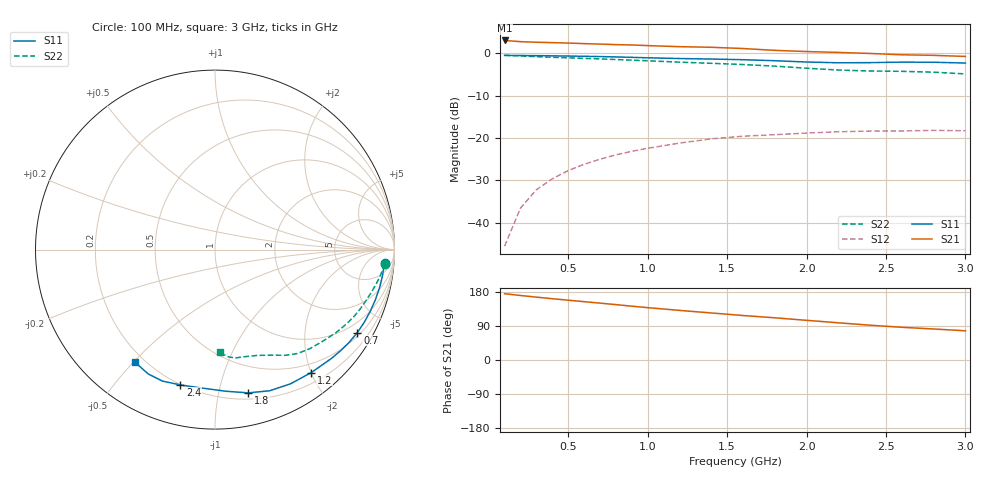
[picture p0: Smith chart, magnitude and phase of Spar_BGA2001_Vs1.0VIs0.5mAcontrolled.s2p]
! Filename: 1_5G1.001
! Title: BGA2001 X0297-20 HFE=80
! Bias: Vce=1V; Ic=.5mA controlled
! Company: NXP Semiconductors NL
! User: Quality&Reliability T&D
! Measure time: 23 Oct 1998 / 08:33:08
#  MHz  S  MA  R 50
! Freq  S11  S21  S12  S22  :
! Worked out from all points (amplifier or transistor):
!   20 points, 100 MHz to 3 GHz, reference 50 ohm
!   highest |S21| = 3.1 dB at 100 MHz (marker M1)
!   |S21| within 3 dB of that: start of sweep to 2.337 GHz
!   unconditionally stable (mu >= 1): start of sweep to 109.8 MHz
!   at 400 MHz: K = 0.26, MSG = 16.1 dB, |S12| = -29.6 dB
!   at 1.2 GHz: K = 0.40, MSG = 11.4 dB, |S12| = -21.2 dB
!   at 3 GHz: K = 0.99, MSG = 8.8 dB, |S12| = -18.3 dB
!   lowest NFmin = 1.33 dB at 1.8 GHz
!   S11 on the Smith chart (normalised r, x): 100 MHz: 12, -17; 700 MHz: 0.61, -3.61; 1.2 GHz: 0.35, -2.00; 1.8 GHz: 0.25, -1.23; 2.4 GHz: 0.20, -0.76; 3 GHz: 0.16, -0.51
100  0.9471 -4.4  1.423 174.9  0.00526 52.8  0.9494 -4.8
200  0.9448 -8.7  1.377 170.3  0.01484 84.0  0.933 -8.9
300  0.9412 -13.1  1.356 165.9  0.02445 80.6  0.9161 -12.5
400  0.9362 -17.4  1.341 161.7  0.03295 77.1  0.9 -15.9
500  0.9309 -21.7  1.326 157.8  0.04113 74.1  0.8861 -19.1
600  0.925 -26.0  1.306 153.9  0.04888 71.1  0.8739 -22.3
700  0.918 -30.2  1.289 150.1  0.05613 68.2  0.8614 -25.3
800  0.9091 -34.5  1.27 146.2  0.06314 65.3  0.8469 -28.3
900  0.8985 -38.8  1.259 142.0  0.06951 62.4  0.8324 -31.3
1000  0.888 -43.1  1.237 138.2  0.07555 59.7  0.8183 -34.3
1200  0.8702 -51.9  1.202 130.9  0.08697 54.3  0.7882 -40.3
1400  0.8579 -60.7  1.182 124.2  0.09768 49.3  0.7641 -46.2
1600  0.8431 -68.9  1.142 117.4  0.105 44.9  0.7394 -51.5
1800  0.8197 -76.9  1.087 111.4  0.1094 41.4  0.7075 -56.4
2000  0.7917 -85.5  1.052 104.7  0.1144 36.7  0.6686 -61.6
2200  0.7749 -95.2  1.027 98.2  0.1185 31.8  0.6362 -67.9
2400  0.7782 -104.3  0.9987 91.8  0.1208 28.0  0.6195 -74.4
2600  0.7889 -111.8  0.9638 86.3  0.1211 26.0  0.614 -79.6
2800  0.7862 -118.3  0.9488 81.8  0.123 23.1  0.6002 -83.4
3000  0.7698 -125.2  0.9212 77.1  0.1217 20.8  0.5725 -87.4
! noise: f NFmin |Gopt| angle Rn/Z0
900  1.46  0.71  23.8  0.95
1000  1.61  0.7  25.8  0.91
1800  1.331  0.622  72.15  0.659
2000  1.625  0.606  84.7  0.598
2200  2.181  0.552  94.89  0.515
2400  2.473  0.577  102.9  0.484
